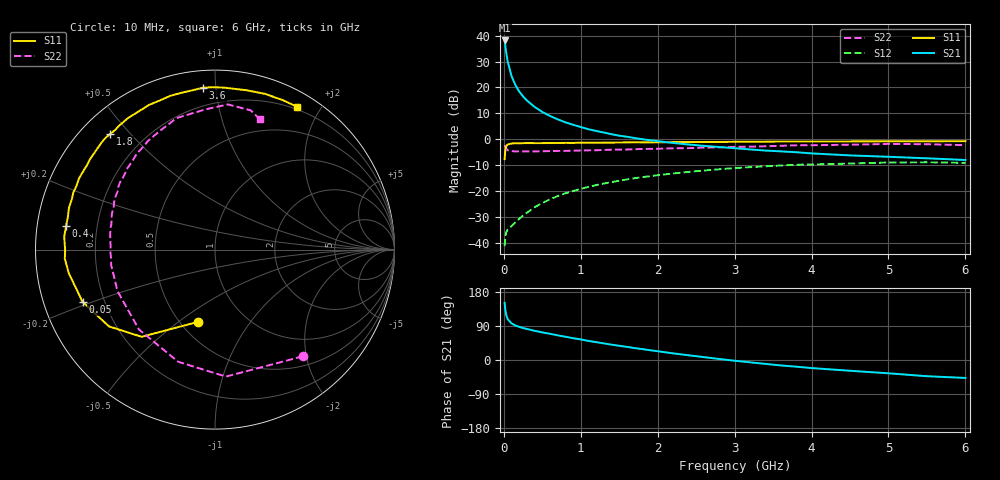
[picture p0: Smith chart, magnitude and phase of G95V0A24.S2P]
! SIEMENS Small Signal Semiconductors
! BFG235
! Si NPN RF Bipolar Junction Transistor in SOT223
! VCE = 5 V  IC = 240 mA
! Common Emitter S-Parameters:  July  1994
# GHz  S  MA  R  50
!  f  S11  S21  S12  S22
! GHz  MAG  ANG  MAG  ANG  MAG  ANG  MAG  ANG
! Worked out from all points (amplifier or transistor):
!   40 points, 10 MHz to 6 GHz, reference 50 ohm
!   highest |S21| = 38.1 dB at 10 MHz (marker M1)
!   |S21| within 3 dB of that: start of sweep to 23.38 MHz
!   unconditionally stable (mu >= 1): 410.9 MHz to 1.537 GHz
!   at 200 MHz: K = 0.85, MSG = 24.6 dB, |S12| = -30.7 dB
!   at 1.5 GHz: K = 1.01, MAG = 8.2 dB, |S12| = -16.0 dB
!   at 6 GHz: K = 0.91, MSG = 0.6 dB, |S12| = -9.1 dB
!   S11 on the Smith chart (normalised r, x): 10 MHz: 0.61, -0.59; 50 MHz: 0.12, -0.19; 400 MHz: 0.09, +0.08; 1.8 GHz: 0.08, +0.44; 3.6 GHz: 0.09, +0.92; 6 GHz: 0.17, +1.72
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0.01  0.4128 -103.0  80.8 150.8  0.0086 59.3  0.7703 -50.5
0.02  0.6351 -130.1  62.42 131.3  0.0134 45.8  0.7102 -85.1
0.03  0.7295 -144.1  48.21 119.8  0.0157 39.2  0.6577 -108.2
0.05  0.7933 -158.5  31.66 107.8  0.018 34.2  0.6146 -133.6
0.1  0.8254 -170.9  16.61 96.6  0.021 39.6  0.5903 -156.9
0.15  0.8384 -176.6  11.13 91.0  0.0248 46.0  0.5821 -166.5
0.2  0.8348 -179.8  8.321 87.5  0.0291 51.3  0.585 -171.6
0.25  0.8385 177.5  6.705 84.3  0.0337 55.0  0.5813 -175.1
0.3  0.8431 175.0  5.597 81.9  0.0381 57.7  0.5826 -178.3
0.4  0.8397 170.8  4.21 77.0  0.0485 60.1  0.5822 177.7
0.5  0.8399 167.3  3.363 72.8  0.0587 61.4  0.5865 174.4
0.7  0.8454 160.6  2.423 65.0  0.0799 61.2  0.5943 168.5
0.9  0.8495 155.4  1.901 57.6  0.0999 58.8  0.6003 163.8
1.1  0.8544 149.0  1.559 50.3  0.1201 56.1  0.6106 159.0
1.4  0.8605 141.8  1.25 40.5  0.1484 50.8  0.6265 152.8
1.8  0.8699 132.2  0.999 28.8  0.1849 43.6  0.6485 144.7
2.2  0.8788 123.4  0.848 17.5  0.2179 36.0  0.6671 136.8
3.2  0.8933 102.1  0.635 -6.1  0.2887 16.6  0.7194 118.2
3.6  0.9043 94.3  0.583 -14.4  0.3108 8.2  0.7459 110.0
4.5  0.905 78.8  0.487 -28.4  0.3391 -8.0  0.783 93.9
5.5  0.9143 65.7  0.428 -42.8  0.3589 -26.0  0.8009 75.6
6  0.9178 60.0  0.397 -47.3  0.3493 -32.8  0.7678 71.0
